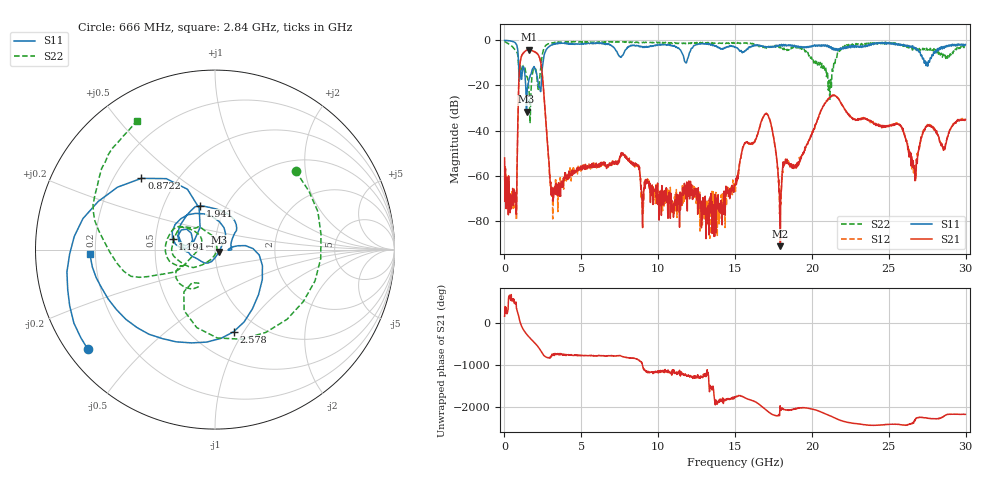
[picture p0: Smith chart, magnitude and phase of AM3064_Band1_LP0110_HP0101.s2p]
# Hz S DB R 50.0
!freq dBS11 angS11 dBS21 angS21 dBS12 angS12 dBS22 angS22
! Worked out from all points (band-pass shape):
!   1600 points, 10 MHz to 29.98 GHz, reference 50 ohm
!   highest |S21| = -4.13 dB at 1.584 GHz (marker M1); lowest = -91.3 dB at 17.95 GHz (marker M2)
!   |S21| within 3 dB of the highest: 1.101 GHz to 2.251 GHz (1.151 GHz wide, 68.7 % of centre)
!   lowest |S11| = -31.6 dB at 1.435 GHz (marker M3), VSWR 1.05, Z = 52.3 - j1.45 ohm
!   |S11| at or under -10 dB: 916.9 MHz to 2.505 GHz (1.588 GHz wide, 92.8 % of centre); 27.39338 GHz to 27.45857 GHz (65.19 MHz wide, 0.238 % of centre); 27.4884 GHz to 27.56252 GHz (74.11 MHz wide, 0.269 % of centre)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
!   |S22| runs from -36.8 to -0.4 dB; largest |S21 - S12| = 0.0076
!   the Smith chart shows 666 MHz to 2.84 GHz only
!   S11 on the Smith chart (normalised r, x): 666 MHz: 0.06, -0.34; 872.2 MHz: 0.31, +0.37; 1.191 GHz: 0.61, +0.08; 1.941 GHz: 0.76, +0.40; 2.578 GHz: 0.77, -0.90; 2.84 GHz: 0.18, -0.02
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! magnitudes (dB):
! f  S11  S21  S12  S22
! 10 MHz  0.0  -52.2  -60.3  -0.4
! 666 MHz  -0.9  -71.2  -70.1  -4.1
! 872.2 MHz  -4.9  -36.0  -36.1  -7.0
! 1.191 GHz  -12.2  -6.0  -5.9  -11.6
! 1.435 GHz  -31.6  -4.4  -4.3  -16.0
! 1.584 GHz  -17.7  -4.1  -4.1  -21.5
! 1.941 GHz  -11.8  -5.1  -5.0  -12.5
! 2.578 GHz  -6.6  -25.1  -25.1  -3.3
! 2.84 GHz  -3.1  -49.9  -49.9  -1.5
! 3.14 GHz  -1.8  -65.5  -79.2  -1.2
! 5.015 GHz  -1.4  -55.9  -57.4  -0.7
! 7.714 GHz  -6.4  -50.0  -50.4  -0.7
! 10 GHz  -2.1  -70.1  -66.5  -0.9
! 15 GHz  -2.9  -64.3  -63.5  -1.4
! 17.03 GHz  -3.0  -32.4  -32.5  -3.5
! 17.95 GHz  -2.3  -91.3  -66.9  -2.8
! 19.99 GHz  -2.9  -41.5  -41.6  -8.4
! 21.4 GHz  -3.6  -24.5  -24.4  -12.4
! 25 GHz  -1.0  -38.2  -37.8  -1.2
! 26.64 GHz  -3.3  -56.5  -58.1  -3.8
! 27.49 GHz  -10.0  -38.2  -37.7  -4.0
! 29.98 GHz  -1.8  -35.1  -35.4  -2.9
